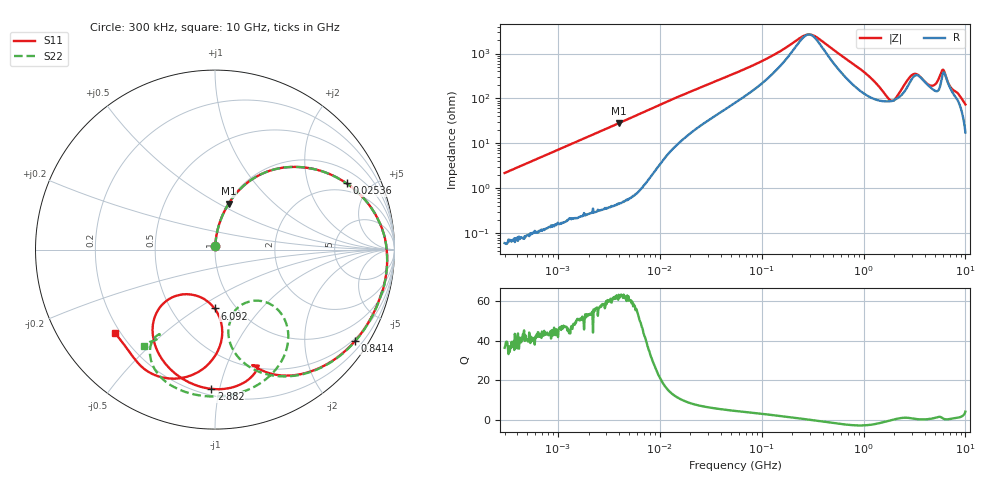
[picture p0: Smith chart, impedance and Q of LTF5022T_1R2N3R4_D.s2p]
! S-Parameter Data Generated by TDK Corporation
! Copyright(C) 2020 TDK Corporation.
! All Rights Reserved.
! TDK P/N: LTF5022T-1R2N3R4-D (Inductor)
! Property: L=1.2uH at 100kHz
! Size(LxWxT): 6.5x5x2.2mm
! Model Type: s2p (Touchstone File Format Version 1.0)
! Frequency: DC=Yes Start=0.3MHz Stop=10000MHz 802points Log-sweep
! Model Generated on Apr. 23, 2020
! Port Assignments:
!  1 ---@@@--- 2
! Applicable Conditions:
!  Temperature = 25 degC
!  DC Bias Current = 0 A
!  Small Signal Operation
! Terms and conditions regarding TDK Simulation Models
! (1)This simulation model is being provided solely for informational purposes. Please refer to the specifications of the products in terms of detailed characteristics of such products.
! (2)In no event shall TDK Corporation of any of its subsidiaries be liable for any loss or damage arising, directly or indirectly,
!  From any information contained in this simulation model, including, but not limited to loss or damages arising from any inaccuracies, omissions or errors in connection with such information.
! (3)Any and all copyrights on this simulation model are owned by TDK Corporation.
!  Duplication or redistribution of this simulation model without prior written permission from TDK Corporation is prohibited.
! (4)This simulation model is subject to any modification or change without any prior notice.
! (5)Neither TDK Corporation nor any of its subsidiaries shall make any warranty, express or implied,
!  Including but not limited to the correctness, implied warranties of merchantability and fitness for a particular purpose with respect to this simulation models.
! (6)The use of this simulation model shall be deemed to have consented to the terms and conditions hereof.
# Hz S MA R 50
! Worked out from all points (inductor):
!   801 points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, 300 kHz to 10 GHz, reference 50 ohm
!   read as one part in series: L = 1.16 uH near 318.3 kHz
!   highest Q = 62.7 at 3.956 MHz (marker M1), where L = 1.13 uH
!   self-resonance near 291.4 MHz
!   S11 on the Smith chart (normalised r, x): 300 kHz: 1.00, +0.04; 25.36 MHz: 1.57, +3.56; 841.4 MHz: 0.43, -3.30; 2.882 GHz: 0.24, -0.94; 6.092 GHz: 0.80, -0.59; 10 GHz: 0.18, -0.35
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300000  0.02196 87.7  0.9992 -1.2  0.9989 -1.3  0.02189 87.3
1713600  0.1203 81.9  0.9905 -7.0  0.9902 -7.0  0.1202 81.9
3956438  0.268 73.4  0.9592 -15.7  0.9592 -15.7  0.2679 73.4
9671944  0.5602 53.2  0.804 -34.3  0.804 -34.3  0.5602 53.2
2.53611e7  0.8206 26.7  0.4662 -55.1  0.4662 -55.1  0.8207 26.7
5.477226e7  0.9138 12.6  0.2519 -64.7  0.2519 -64.7  0.9139 12.5
2.569609e8  0.963 -6.8  0.03894 -28.1  0.03893 -28.1  0.9633 -7.1
3.126428e8  0.9633 -9.7  0.03686 2.8  0.03685 2.9  0.9636 -10.1
8.414386e8  0.9314 -33.2  0.1597 37.4  0.1596 37.5  0.9288 -35.0
1.35547e9  0.842 -55.5  0.3026 9.3  0.3023 9.4  0.8049 -61.4
1.767019e9  0.7187 -69.0  0.4013 -25.8  0.4015 -25.7  0.5495 -80.3
2.020878e9  0.6912 -69.3  0.4039 -51.6  0.4043 -51.5  0.3557 -71.5
2.23379e9  0.7146 -71.4  0.355 -72.9  0.3552 -72.9  0.3881 -47.7
2.53795e9  0.7655 -79.6  0.2478 -94.9  0.2471 -95.2  0.5936 -47.2
2.882439e9  0.7761 -91.5  0.1537 -102.7  0.1514 -103.0  0.7367 -61.1
3.34571e9  0.7336 -106.0  0.1086 -92.5  0.1056 -91.3  0.8055 -78.2
4.34106e9  0.5665 -127.9  0.112 -95.5  0.1134 -92.6  0.8095 -102.1
5.284132e9  0.3426 -130.7  0.08419 -115.4  0.09144 -112.3  0.7544 -115.7
6.091595e9  0.3278 -90.4  0.05187 -87.1  0.05848 -96.7  0.6653 -123.0
6.737565e9  0.5437 -87.4  0.1047 -76.4  0.09711 -81.9  0.592 -124.4
7.652089e9  0.7422 -105.1  0.1514 -110.5  0.1392 -110.4  0.5642 -123.1
1e10  0.7232 -140.2  0.1817 -167.5  0.1823 -165.3  0.6695 -126.3
